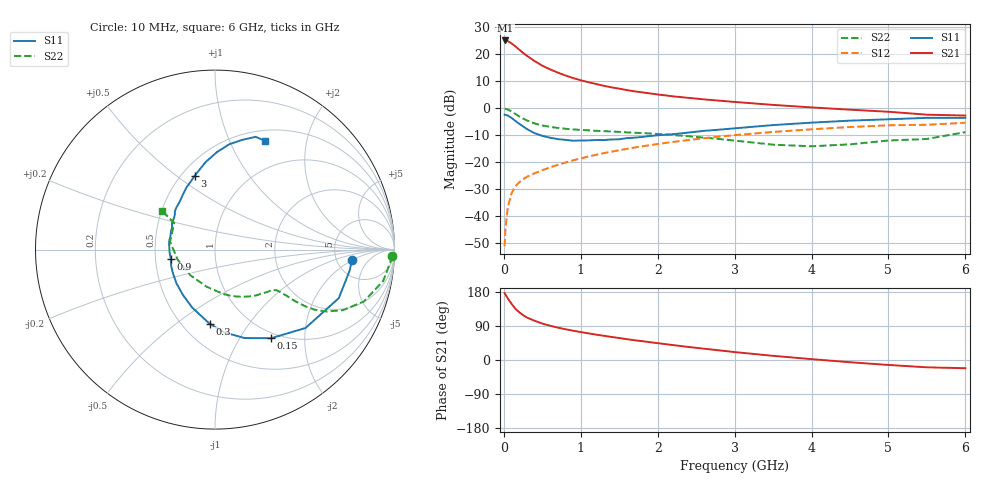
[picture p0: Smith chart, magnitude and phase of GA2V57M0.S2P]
! Infineon Technologies  Discrete & RF Semiconductors
! BF775
! Si NPN RF Bipolar Junction Transistor in SOT23
! VCE = 2.5 V  IC = 7 mA
! Common Emitter S-Parameters:  May  1996
# GHz  S  MA  R  50
!  f  S11  S21  S12  S22
! GHz  MAG  ANG  MAG  ANG  MAG  ANG  MAG  ANG
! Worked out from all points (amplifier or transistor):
!   36 points, 10 MHz to 6 GHz, reference 50 ohm
!   highest |S21| = 25.2 dB at 20 MHz (marker M1)
!   |S21| within 3 dB of that: start of sweep to 183.5 MHz
!   unconditionally stable (mu >= 1): 667.4 MHz to 3.613 GHz
!   at 250 MHz: K = 0.58, MSG = 23.4 dB, |S12| = -26.2 dB
!   at 1.4 GHz: K = 1.13, MAG = 9.7 dB, |S12| = -16.0 dB
!   at 6 GHz: K = 0.97, MSG = 1.3 dB, |S12| = -5.3 dB
!   S11 on the Smith chart (normalised r, x): 10 MHz: 6.97, -1.98; 150 MHz: 0.92, -1.38; 300 MHz: 0.67, -0.67; 900 MHz: 0.60, -0.07; 3 GHz: 0.58, +0.58; 6 GHz: 0.63, +1.37
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0.01  0.7658 -4.4  18.06 176.6  0.0028 90.5  0.9871 -2.1
0.02  0.7592 -8.9  18.14 172.8  0.0056 85.0  0.9785 -4.3
0.05  0.7409 -21.4  17.7 162.9  0.0144 80.1  0.9531 -10.6
0.1  0.6672 -40.9  15.97 148.2  0.0267 70.8  0.8785 -19.2
0.15  0.5847 -57.6  14.1 135.1  0.0359 64.8  0.7895 -25.3
0.2  0.5195 -71.5  12.26 126.0  0.0428 61.4  0.7117 -29.0
0.25  0.4649 -83.4  10.67 118.3  0.0487 59.4  0.6485 -31.1
0.3  0.4139 -94.2  9.414 112.1  0.0539 58.3  0.5981 -32.1
0.4  0.3473 -111.4  7.534 103.5  0.0628 57.9  0.5266 -32.8
0.5  0.3094 -125.3  6.18 96.2  0.0715 58.6  0.4823 -32.8
0.6  0.286 -138.4  5.29 90.5  0.0806 59.1  0.455 -32.9
0.7  0.2698 -149.8  4.61 85.5  0.0897 59.7  0.4349 -33.0
0.9  0.2519 -167.5  3.651 77.3  0.109 60.2  0.4074 -33.7
1.1  0.2554 176.3  3.053 70.3  0.1284 60.1  0.3922 -35.7
1.3  0.2588 163.9  2.62 63.9  0.1484 59.3  0.3782 -38.0
1.6  0.2817 148.3  2.179 54.9  0.1778 57.7  0.3591 -42.5
2.2  0.3323 126.2  1.672 39.3  0.2391 52.5  0.3208 -54.6
3  0.4267 105.4  1.317 20.9  0.3196 43.4  0.2531 -78.8
3.5  0.4905 96.1  1.16 11.0  0.3656 37.0  0.2126 -102.3
4.5  0.5927 82.2  0.946 -5.9  0.4513 23.8  0.2156 -164.8
5.5  0.6678 70.2  0.765 -19.3  0.4977 9.1  0.2713 146.9
6  0.6666 65.3  0.736 -21.7  0.5414 5.1  0.3627 143.9
